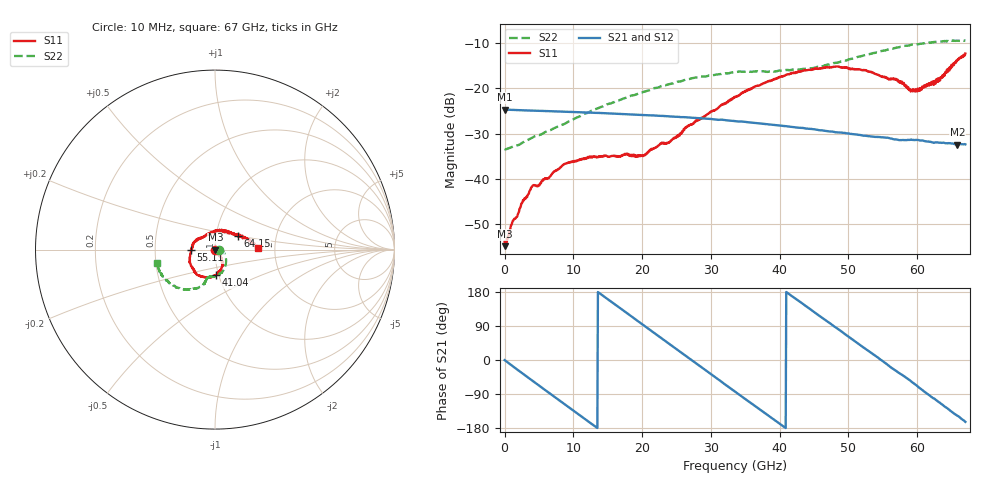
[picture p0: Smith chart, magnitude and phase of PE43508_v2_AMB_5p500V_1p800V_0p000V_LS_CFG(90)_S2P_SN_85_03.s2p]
!Keysight Technologies,N5227A,US51270237,A.10.43.00
!Date: Wednesday, August 22, 2018 17:16:03
!Correction: S11(Full 2 Port(1,3))
!S31(Full 2 Port(1,3))
!S13(Full 2 Port(1,3))
!S33(Full 2 Port(1,3))
!S2P File: Measurements: S11, S31, S13, S33:
# Hz S  dB  R 50
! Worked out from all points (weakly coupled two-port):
!   801 points, 10 MHz to 67 GHz, reference 50 ohm
!   highest |S21| = -24.73 dB at 10 MHz (marker M1); lowest = -32.4 dB at 65.83 GHz (marker M2)
!   lowest |S11| = -54.8 dB at 93.74 MHz (marker M3), VSWR 1.00, Z = 50.2 - j0.00612 ohm
!   |S11| at or under -10 dB: start of sweep to end of sweep
!   |S22| runs from -33.5 to -9.5 dB; largest |S21 - S12| = 0.00028
!   S11 on the Smith chart (normalised r, x): 10 MHz: 1.00, -0.00; 41.04 GHz: 0.98, -0.28; 55.11 GHz: 0.76, -0.00; 64.15 GHz: 1.27, +0.19; 67 GHz: 1.63, +0.03
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1e7  -53.79 -9.5  -24.73 -0.2  -24.72 -0.2  -33.43 -0.6
9.37375e7  -54.79 -1.9  -24.74 -1.4  -24.75 -1.4  -33.48 0.3
4.286875e8  -52.97 -7.9  -24.76 -6.0  -24.77 -6.0  -33.36 1.6
1.182325e9  -49.26 -22.1  -24.81 -16.3  -24.81 -16.3  -32.88 2.8
4.0294e9  -41.59 -53.3  -24.96 -54.4  -24.97 -54.4  -30.90 1.4
8.7187e9  -36.72 -83.5  -25.20 -116.5  -25.20 -116.5  -27.89 -9.1
1.123082e10  -35.57 -88.7  -25.34 -149.7  -25.34 -149.7  -25.96 -17.7
2.002326e10  -34.81 -76.0  -25.91 94.2  -25.90 94.2  -20.92 -46.6
2.236791e10  -32.63 -65.4  -26.10 63.3  -26.10 63.3  -19.83 -54.8
2.395892e10  -31.91 -58.0  -26.23 42.4  -26.23 42.4  -19.12 -59.7
2.655479e10  -28.49 -54.8  -26.45 8.2  -26.45 8.2  -18.07 -68.2
3.3505e10  -22.01 -60.2  -27.27 -83.5  -27.26 -83.5  -16.50 -90.1
4.104138e10  -17.02 -86.9  -28.40 178.3  -28.40 178.3  -16.00 -102.5
4.472582e10  -15.93 -105.8  -29.02 130.3  -29.01 130.4  -15.63 -104.9
4.841028e10  -15.25 -125.7  -29.76 82.6  -29.76 82.5  -14.41 -106.9
5.510928e10  -17.50 -179.6  -30.88 -4.8  -30.85 -5.1  -11.79 -121.1
5.586291e10  -18.11 172.6  -30.99 -15.4  -30.97 -15.7  -11.45 -123.6
6.004979e10  -20.15 107.3  -31.41 -69.4  -31.42 -69.8  -10.39 -138.2
6.29806e10  -17.88 54.0  -31.94 -109.0  -31.98 -109.5  -9.87 -149.9
6.415292e10  -16.69 30.6  -32.16 -124.9  -32.21 -125.1  -9.68 -154.2
6.582768e10  -13.87 14.7  -32.43 -147.1  -32.50 -147.4  -9.60 -160.8
6.7e10  -12.39 1.8  -32.38 -163.3  -32.44 -163.4  -9.55 -167.0
